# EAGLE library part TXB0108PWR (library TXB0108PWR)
8-Bit Bidirectional Voltage-Level Shifter with Auto Direction Sensing and +/-15-kV ESD Protect Source: Datasheet
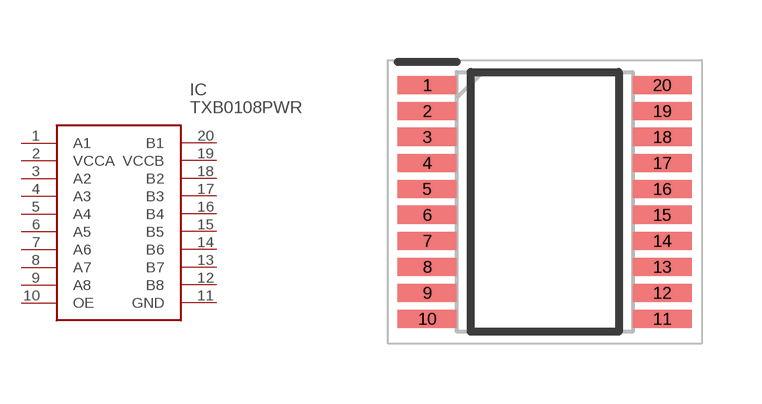
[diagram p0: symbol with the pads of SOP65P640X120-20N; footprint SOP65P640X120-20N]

Designator prefix IC

## TXB0108PWR (Description: 8-Bit Bidirectional Voltage-Level Shifter with Auto Direction Sensing and +/-15-kV ESD Protect; Height: 1.2mm; Manufacturer_Name: Texas Instruments; Manufacturer_Part_Number: TXB0108PWR; Mouser_Part_Number: 595-TXB0108PWR; Mouser_Price-Stock: https://www.mouser.co.uk/ProductDetail/Texas-Instruments/TXB0108PWR/?qs=oFXvjAmG9EgEUWGWzOVFCA%3D%3D)  [SOP65P640X120-20N]
1  A1
2  VCCA
3  A2
4  A3
5  A4
6  A5
7  A6
8  A7
9  A8
10  OE
11  GND
12  B8
13  B7
14  B6
15  B5
16  B4
17  B3
18  B2
19  VCCB
20  B1

## Footprint SOP65P640X120-20N (pad centres in mm)
PW (R-PDSO-G20)
smd 1.475 x 0.45: 1 -2.938,2.925; 2 -2.938,2.275; 3 -2.938,1.625; 4 -2.938,0.975; 5 -2.938,0.325; 6 -2.938,-0.325; 7 -2.938,-0.975; 8 -2.938,-1.625; 9 -2.938,-2.275; 10 -2.938,-2.925; 11 2.938,-2.925; 12 2.938,-2.275; 13 2.938,-1.625; 14 2.938,-0.975; 15 2.938,-0.325; 16 2.938,0.325; 17 2.938,0.975; 18 2.938,1.625; 19 2.938,2.275; 20 2.938,2.925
